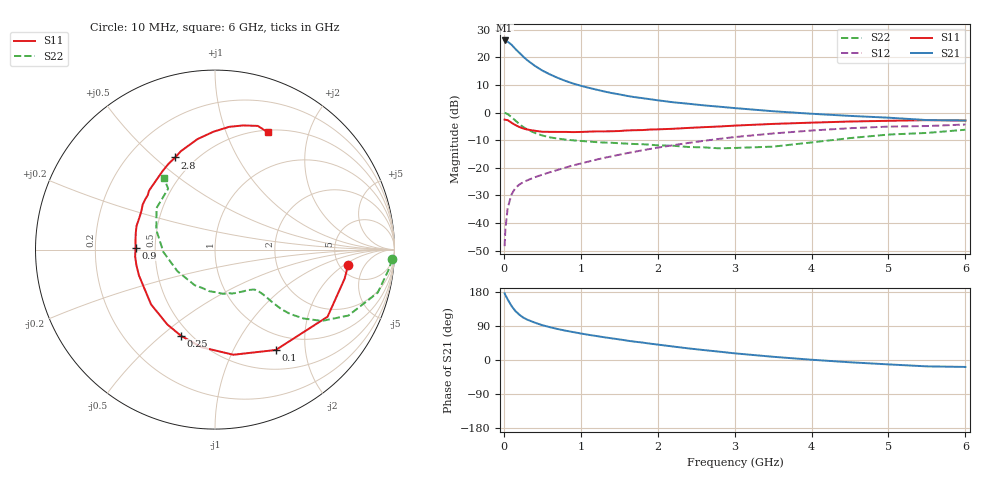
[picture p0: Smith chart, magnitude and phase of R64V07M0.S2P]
! SIEMENS Small Signal Semiconductors
! BFR193
! Si NPN RF Bipolar Junction Transistor in SOT23
! VCE = 4 V  IC = 7 mA
! Common Emitter S-Parameters:  May  1996
# GHz  S  MA  R  50
!  f  S11  S21  S12  S22
! GHz  MAG  ANG  MAG  ANG  MAG  ANG  MAG  ANG
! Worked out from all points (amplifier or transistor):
!   36 points, 10 MHz to 6 GHz, reference 50 ohm
!   highest |S21| = 26.1 dB at 10 MHz (marker M1)
!   |S21| within 3 dB of that: start of sweep to 147.9 MHz
!   unconditionally stable (mu >= 1): 823 MHz to 2.006 GHz
!   at 250 MHz: K = 0.53, MSG = 22.8 dB, |S12| = -25.3 dB
!   at 1.4 GHz: K = 1.05, MAG = 10.0 dB, |S12| = -15.9 dB
!   at 6 GHz: K = 0.95, MSG = 0.7 dB, |S12| = -4.3 dB
!   lowest NFmin = 1.20 dB at 450 MHz
!   S11 on the Smith chart (normalised r, x): 10 MHz: 6.03, -2.28; 100 MHz: 0.76, -1.49; 250 MHz: 0.45, -0.58; 900 MHz: 0.39, +0.01; 2.8 GHz: 0.39, +0.58; 6 GHz: 0.53, +1.41
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0.01  0.7472 -6.4  20.25 176.0  0.0038 91.7  0.9875 -3.1
0.02  0.74 -12.7  19.96 171.4  0.0076 83.0  0.9769 -6.1
0.05  0.7301 -30.8  19.22 159.7  0.0187 76.1  0.938 -14.8
0.1  0.6538 -58.8  16.98 142.6  0.033 65.6  0.8291 -26.3
0.15  0.5947 -80.1  14.23 129.3  0.043 57.7  0.7163 -33.7
0.2  0.549 -97.8  12.15 119.8  0.0495 54.0  0.6248 -37.9
0.25  0.5161 -111.6  10.39 112.3  0.0545 52.0  0.5501 -40.6
0.3  0.4943 -122.6  8.983 106.8  0.0589 51.5  0.4979 -41.9
0.4  0.4692 -139.4  7.075 98.8  0.0672 52.0  0.4299 -42.6
0.5  0.4489 -151.5  5.774 91.9  0.075 53.7  0.3841 -42.8
0.6  0.4474 -161.2  4.913 86.5  0.0831 55.2  0.3555 -43.2
0.7  0.4465 -168.6  4.26 81.7  0.0916 56.4  0.3383 -43.7
0.9  0.4427 178.5  3.362 73.7  0.1104 58.5  0.3142 -45.3
1.1  0.4511 168.1  2.82 66.6  0.1295 60.0  0.299 -48.6
1.3  0.4565 159.2  2.421 60.2  0.1508 60.3  0.2864 -52.3
1.6  0.4746 148.1  2.008 51.2  0.1837 59.9  0.2739 -59.8
2.2  0.5086 129.4  1.538 35.6  0.2563 55.8  0.2509 -79.5
2.8  0.5592 113.4  1.279 22.0  0.334 48.9  0.2252 -108.6
3.5  0.6234 99.0  1.058 8.5  0.4183 38.5  0.2416 -150.2
4.5  0.6886 83.4  0.871 -6.0  0.5213 22.7  0.345 161.4
5.5  0.7293 70.9  0.731 -16.8  0.5703 6.4  0.4278 127.6
6  0.7165 65.7  0.72 -18.3  0.6082 1.6  0.489 125.5
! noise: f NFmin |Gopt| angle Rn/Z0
0.45  1.2  0.24  125  0.12
0.9  1.25  0.36  154  0.11
1.8  2  0.55  -156  0.13
